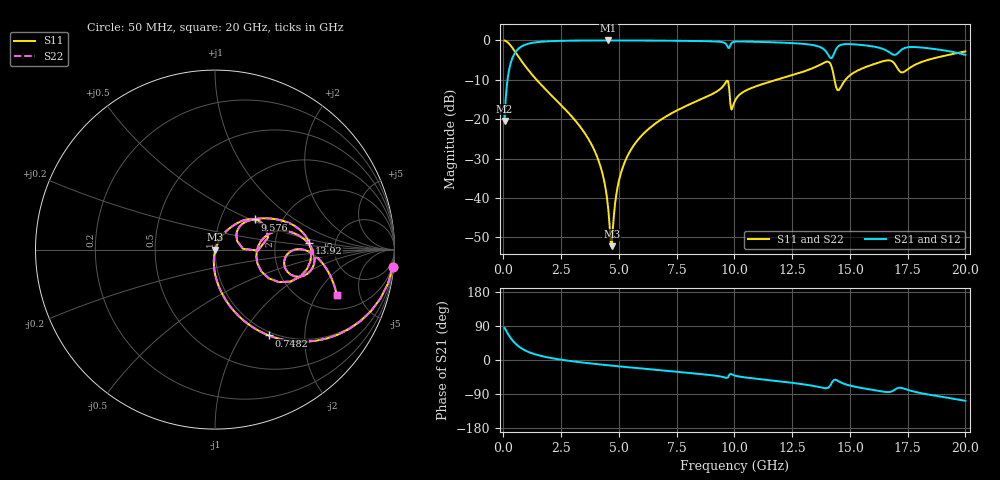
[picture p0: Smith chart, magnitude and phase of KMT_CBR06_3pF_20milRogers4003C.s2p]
! Data measured by Modelithics Inc. support@modelithics.com 813-866-6335
! KEMET CBR0603 3pF, Pad Width= 0.851mm, Pad Length= 0.64mm, Pad Gap= 0.62mm, 20mil Rogers 4003C substrate Data, January 2022
# hz S ma R 50
! 2 Port Network Data from SP1.SP block
! freq  magS11  angS11  magS21  angS21  magS12  angS12  magS22  angS22
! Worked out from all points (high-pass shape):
!   401 points, 50 MHz to 20 GHz, reference 50 ohm
!   highest |S21| = -0.02 dB at 4.539 GHz (marker M1); lowest = -20.5 dB at 50 MHz (marker M2)
!   |S21| within 3 dB of the highest: 519.5 MHz to 13.99 GHz (13.47 GHz wide, 186 % of centre); 17.11 GHz to 19.53 GHz (2.418 GHz wide, 13.2 % of centre)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
!   lowest |S11| = -52.2 dB at 4.688 GHz (marker M3), VSWR 1.00, Z = 50.2 + j0.0264 ohm
!   |S11| at or under -10 dB: 1.433 GHz to 11.83 GHz (10.39 GHz wide, 157 % of centre); 14.33 GHz to 14.81 GHz (475.7 MHz wide, 3.26 % of centre)
!   |S22| runs from -52.2 to 0.0 dB; largest |S21 - S12| = 0
!   S11 on the Smith chart (normalised r, x): 50 MHz: 1, -20; 748.2 MHz: 0.95, -1.33; 9.576 GHz: 1.46, +0.53; 13.92 GHz: 3.19, +0.32; 20 GHz: 2.83, -3.03
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5e7  0.9955 -5.6  0.09481 84.4  0.09481 84.4  0.9955 -5.6
2.99375e8  0.8675 -30.7  0.4966 59.2  0.4966 59.2  0.8675 -30.7
7.4825e8  0.5645 -57.9  0.8244 32.0  0.8244 32.0  0.5645 -57.9
1.596125e9  0.2804 -78.5  0.9585 11.2  0.9585 11.2  0.2804 -78.5
3.391625e9  0.07518 -95.0  0.9951 -6.4  0.9951 -6.4  0.07518 -95.0
4.189625e9  0.02573 -97.0  0.9974 -11.8  0.9974 -11.8  0.02573 -97.0
4.53875e9  0.007179 -85.8  0.9976 -14.0  0.9976 -14.0  0.007179 -85.8
4.688375e9  0.002442 6.2  0.9976 -14.9  0.9976 -14.9  0.002442 6.2
4.987625e9  0.01592 64.8  0.9973 -16.7  0.9973 -16.7  0.01592 64.8
5.286875e9  0.03014 66.9  0.9969 -18.4  0.9969 -18.4  0.03014 66.9
6.73325e9  0.09482 61.6  0.9924 -26.7  0.9924 -26.7  0.09482 61.6
9.576125e9  0.2784 37.2  0.9281 -46.1  0.9281 -46.1  0.2784 37.2
1.0025e10  0.1712 41.7  0.9639 -41.2  0.9639 -41.2  0.1712 41.7
1.336662e10  0.4412 19.4  0.8751 -67.8  0.8751 -67.8  0.4412 19.4
1.391525e10  0.5268 3.9  0.749 -74.3  0.749 -74.3  0.5268 3.9
1.42145e10  0.4558 -23.0  0.5976 -60.2  0.5976 -60.2  0.4558 -23.0
1.451375e10  0.2336 -1.0  0.8474 -56.1  0.8474 -56.1  0.2336 -1.0
1.54115e10  0.4246 13.7  0.8793 -72.9  0.8793 -72.9  0.4246 13.7
1.670825e10  0.5571 -8.5  0.7051 -84.4  0.7051 -84.4  0.5571 -8.5
1.725688e10  0.391 -9.2  0.7683 -74.0  0.7683 -74.0  0.391 -9.2
1.805488e10  0.5255 -1.4  0.8133 -87.3  0.8133 -87.3  0.5255 -1.4
2e10  0.7245 -20.5  0.6538 -107.7  0.6538 -107.7  0.7245 -20.5
